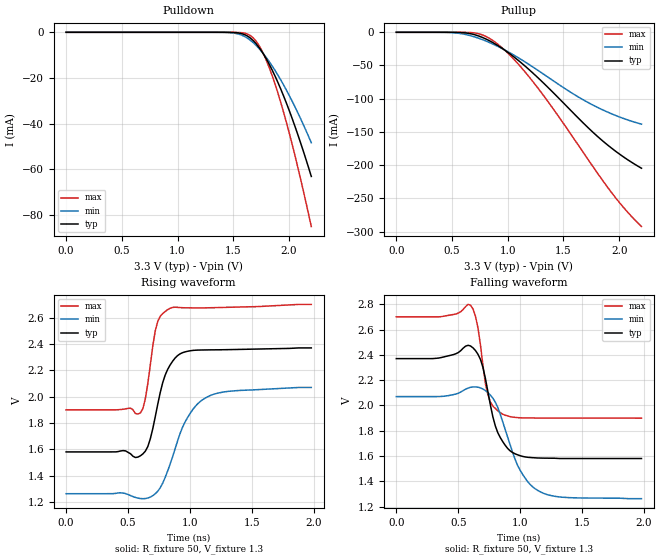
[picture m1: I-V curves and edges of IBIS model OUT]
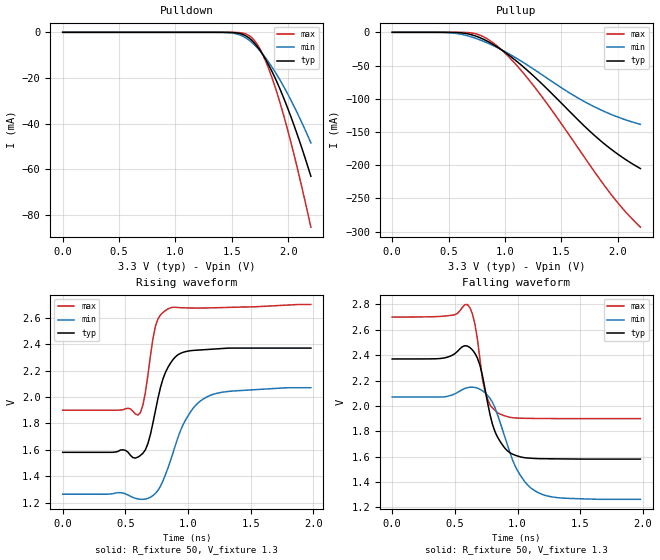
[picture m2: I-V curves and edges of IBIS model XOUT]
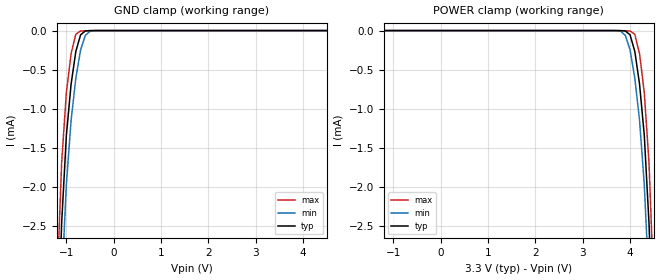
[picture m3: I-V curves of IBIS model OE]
[IBIS Ver]   3.2
[Comment Char]   |_char
[File name]   vg7050ecn_pecl.ibs
[File Rev]   1.2
[Date]   2014/05/08 11:06:20
[Source]
[Notes]
[Disclaimer]
Seiko Epson Corporation makes no warranty with respect to the information
contained herein.
[Copyright]
Copyright(C) 2013, Seiko Epson Corporation. All rights reserved.
[Component]   VG7050ECN_PECL
Si_location Pin
Timing_location Pin
[Manufacturer]   Seiko Epson Corporation
[Package]
R_pkg   0.048   NA   NA
L_pkg   0.48n   NA   NA
C_pkg   0.21p   NA   NA
[Pin] signal_name   model_name   R_pin   L_pin   C_pin
1   GND   GND
2   OE   OE
3   GND   GND
4   OUT   OUT   0.048   0.48n   0.21p
5   XOUT   XOUT   0.048   0.48n   0.21p
6   VCC   POWER
[Diff Pin] inv_pin vdiff   tdelay_typ
4   5   0   0
| Models and submodels in the file (3): OUT (Output_ECL), XOUT (Output_ECL), OE (Input)
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[Model]   OUT
Model_type Output_ECL
Enable Active-High
Polarity Non-Inverting
Vref=1.3
Vmeas=1.97
Rref=50
Cref=0
C_comp   0.121p   0.121p   0.121p
[Temperature Range] 25   85   -40
[Voltage Range]   3.3   2.97   3.63
[Pullup Reference]  3.3   2.97   3.63
[Pulldown Reference]3.3   2.97   3.63
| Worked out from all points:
|   falling waveform, R_fixture 50, V_fixture 1.3: 20-80 % time 125ps typ, 194ps min, 77.9ps max; typ from 2.37 V to 1.58 V
|   rising waveform, R_fixture 50, V_fixture 1.3: 20-80 % time 128ps typ, 213ps min, 78.2ps max; typ from 1.58 V to 2.37 V
[Pullup]
0V        13.3pA     24.45pA    14.68pA
450mV     -11.35uA   -201uA     -118.2nA
625mV     -1.032mA   -3.445mA   -110.4uA
775mV     -7.905mA   -11.2mA    -4.093mA
900mV     -18.82mA   -20.37mA   -16.51mA
1.05V     -36.35mA   -33.86mA   -39.73mA
1.225V    -61.27mA   -52.18mA   -74.11mA
1.375V    -85.3mA    -69.17mA   -107.6mA
1.575V    -119.3mA   -91.41mA   -155.6mA
1.825V    -159.7mA   -114.7mA   -216.8mA
2.025V    -186.1mA   -128.9mA   -261mA
2.2V      -204.7mA   -138.3mA   -292.5mA
[Pulldown]
0V        13.4pA     18.15pA    14.74pA
1.45V     -21.86uA   -105.5uA   -1.875uA
1.575V    -583.5uA   -1.232mA   -181.1uA
1.675V    -3.44mA    -4.369mA   -2.266mA
1.725V    -6.233mA   -6.79mA    -5.305mA
1.775V    -9.869mA   -9.696mA   -9.887mA
1.825V    -14.23mA   -13.03mA   -15.77mA
1.9V      -21.93mA   -18.73mA   -26.55mA
1.975V    -30.82mA   -25.19mA   -39.2mA
2.05V     -40.74mA   -32.33mA   -53.34mA
2.125V    -51.56mA   -40.08mA   -68.73mA
2.2V      -63.16mA   -48.39mA   -85.12mA
[Falling Waveform]
R_fixture=50
V_fixture=1.3
V_fixture_min=0.97
V_fixture_max=1.63
0s        2.37V      2.07V      2.7V
360ps     2.378V     2.071V     2.701V
600ps     2.47V      2.143V     2.792V
660ps     2.404V     2.144V     2.611V
740ps     2.108V     2.102V     2.083V
800ps     1.838V     2.026V     1.977V
860ps     1.714V     1.869V     1.931V
1ns       1.603V     1.489V     1.903V
1.16ns    1.585V     1.32V      1.901V
1.98ns    1.581V     1.264V     1.9V
[Rising Waveform]
R_fixture=50
V_fixture=1.3
V_fixture_min=0.97
V_fixture_max=1.63
0s        1.581V     1.264V     1.9V
600ps     1.552V     1.227V     1.877V
660ps     1.622V     1.231V     2.1V
700ps     1.757V     1.249V     2.384V
740ps     1.942V     1.282V     2.571V
780ps     2.106V     1.344V     2.631V
840ps     2.241V     1.488V     2.671V
960ps     2.34V      1.807V     2.674V
1.14ns    2.355V     1.998V     2.674V
1.98ns    2.37V      2.07V      2.7V
[Ramp]
R_load=50
dV/dt_r   4.734E-1/1.281E-10   4.836E-1/2.130E-10   4.800E-1/7.825E-11
dV/dt_f   4.734E-1/1.246E-10   4.836E-1/1.945E-10   4.800E-1/7.787E-11
|[End   OUT
[Model]   XOUT
Model_type Output_ECL
Enable Active-High
Polarity Inverting
Vref=1.3
Vmeas=1.97
Rref=50
Cref=0
C_comp   0.121p   0.121p   0.121p
[Temperature Range] 25   85   -40
[Voltage Range]   3.3   2.97   3.63
[Pullup Reference]  3.3   2.97   3.63
[Pulldown Reference]3.3   2.97   3.63
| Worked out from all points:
|   falling waveform, R_fixture 50, V_fixture 1.3: 20-80 % time 125ps typ, 194ps min, 81.3ps max; typ from 2.37 V to 1.58 V
|   rising waveform, R_fixture 50, V_fixture 1.3: 20-80 % time 128ps typ, 211ps min, 77.6ps max; typ from 1.58 V to 2.37 V
[Pullup]
0V        13.43pA    22.76pA    14.86pA
450mV     -11.33uA   -200.7uA   -117.9nA
625mV     -1.031mA   -3.444mA   -110.2uA
775mV     -7.908mA   -11.2mA    -4.093mA
900mV     -18.85mA   -20.38mA   -16.53mA
1.05V     -36.41mA   -33.9mA    -39.82mA
1.225V    -61.4mA    -52.25mA   -74.33mA
1.375V    -85.49mA   -69.28mA   -108mA
1.575V    -119.6mA   -91.55mA   -156.2mA
1.825V    -160mA     -114.8mA   -217.6mA
2.025V    -186.4mA   -129.1mA   -261.8mA
2.2V      -205.1mA   -138.5mA   -293.3mA
[Pulldown]
0V        13.43pA    17.73pA    14.89pA
1.45V     -22.1uA    -104.8uA   -1.866uA
1.575V    -584.4uA   -1.227mA   -180.6uA
1.675V    -3.434mA   -4.36mA    -2.263mA
1.725V    -6.22mA    -6.781mA   -5.303mA
1.775V    -9.847mA   -9.688mA   -9.891mA
1.825V    -14.2mA    -13.02mA   -15.79mA
1.9V      -21.88mA   -18.73mA   -26.6mA
1.975V    -30.76mA   -25.2mA    -39.28mA
2.05V     -40.66mA   -32.35mA   -53.48mA
2.125V    -51.47mA   -40.12mA   -68.92mA
2.2V      -63.07mA   -48.44mA   -85.38mA
[Falling Waveform]
R_fixture=50
V_fixture=1.3
V_fixture_min=0.97
V_fixture_max=1.63
0s        2.37V      2.07V      2.7V
480ps     2.4V       2.087V     2.715V
600ps     2.472V     2.144V     2.799V
660ps     2.414V     2.145V     2.644V
740ps     2.135V     2.104V     2.116V
800ps     1.854V     2.028V     1.984V
880ps     1.692V     1.812V     1.928V
1ns       1.605V     1.489V     1.904V
1.16ns    1.585V     1.319V     1.901V
1.98ns    1.581V     1.264V     1.9V
[Rising Waveform]
R_fixture=50
V_fixture=1.3
V_fixture_min=0.97
V_fixture_max=1.63
0s        1.581V     1.264V     1.9V
460ps     1.598V     1.275V     1.901V
620ps     1.557V     1.226V     1.88V
680ps     1.648V     1.232V     2.165V
740ps     1.897V     1.271V     2.536V
800ps     2.137V     1.365V     2.639V
860ps     2.256V     1.518V     2.675V
980ps     2.343V     1.825V     2.674V
1.14ns    2.359V     1.995V     2.674V
1.98ns    2.37V      2.07V      2.7V
[Ramp]
R_load=50
dV/dt_r   4.734E-1/1.284E-10   4.836E-1/2.113E-10   4.800E-1/7.762E-11
dV/dt_f   4.734E-1/1.249E-10   4.836E-1/1.942E-10   4.800E-1/8.127E-11
|[End   XOUT
[Model]   OE
Model_type Input
Vinh=2.31
Vinl=0.99
C_comp   1p   1p   1p
[Temperature Range] 25   85   -40
[Voltage Range]   3.3   2.97   3.63
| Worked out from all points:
|   GND clamp passes 1 mA (typ) near -0.95 V on its own axis
[GND Clamp]
-3.3V     -51.91mA   -51.41mA   -52.45mA
-1.2V     -4.172mA   -5.037mA   -3.304mA
-1.1V     -2.464mA   -3.264mA   -1.692mA
-1V       -1.336mA   -1.965mA   -792.1uA
-900mV    -683.3uA   -1.145mA   -293.8uA
-800mV    -265.5uA   -607.4uA   -46.87uA
-700mV    -54.67uA   -246.7uA   -5.009uA
-600mV    -4.978uA   -61.64uA   -2.11uA
-500mV    -569nA     -7.808uA   -818.7nA
-400mV    -83.43nA   -552.6nA   -153.5nA
6.6V      224.3pA    337.7pA    197.1pA
[POWER Clamp]
-3.3V     224.5pA    337.7pA    197pA
3.7V      -83.43nA   -552.6nA   -153.5nA
3.8V      -569nA     -7.808uA   -818.7nA
3.9V      -4.978uA   -61.64uA   -2.11uA
4V        -54.67uA   -246.7uA   -5.009uA
4.1V      -265.5uA   -607.4uA   -46.87uA
4.2V      -683.3uA   -1.145mA   -293.8uA
4.3V      -1.336mA   -1.965mA   -792.1uA
4.4V      -2.464mA   -3.264mA   -1.692mA
4.5V      -4.172mA   -5.037mA   -3.304mA
6.6V      -51.91mA   -51.41mA   -52.45mA
